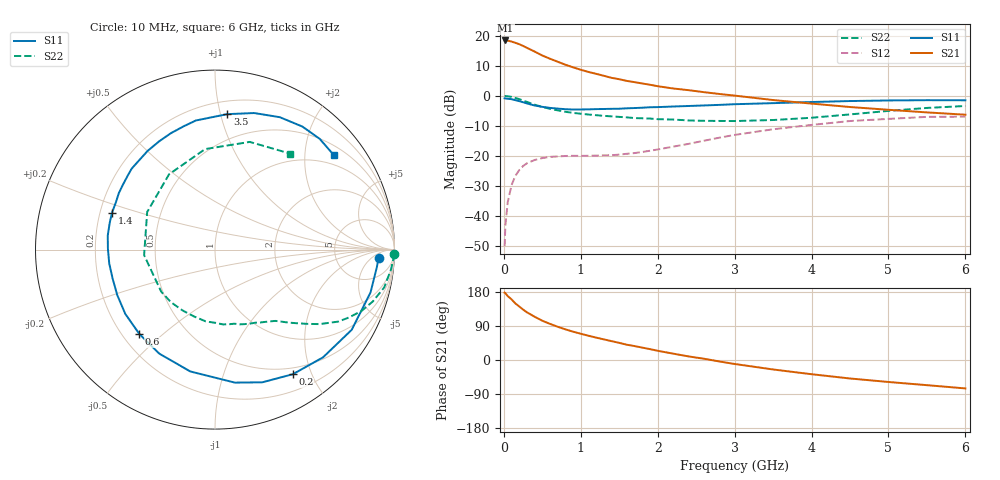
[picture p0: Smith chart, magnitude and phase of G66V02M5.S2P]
! SIEMENS Small Signal Semiconductors
! BFG193
! Si NPN RF Bipolar Junction Transistor in SOT223
! VCE = 6 V  IC = 2.5 mA
! Common Emitter S-Parameters:  August  1996
# GHz  S  MA  R  50
!  f  S11  S21  S12  S22
! GHz  MAG  ANG  MAG  ANG  MAG  ANG  MAG  ANG
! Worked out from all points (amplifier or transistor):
!   36 points, 10 MHz to 6 GHz, reference 50 ohm
!   highest |S21| = 18.5 dB at 20 MHz (marker M1)
!   |S21| within 3 dB of that: start of sweep to 343.2 MHz
!   unconditionally stable (mu >= 1): 1.33 GHz to 2.536 GHz
!   at 250 MHz: K = 0.20, MSG = 20.1 dB, |S12| = -23.4 dB
!   at 1.4 GHz: K = 1.05, MAG = 11.5 dB, |S12| = -19.8 dB
!   at 6 GHz: K = 0.93, MSG = 0.3 dB, |S12| = -6.9 dB
!   S11 on the Smith chart (normalised r, x): 10 MHz: 16, -9; 200 MHz: 0.41, -1.73; 600 MHz: 0.27, -0.42; 1.4 GHz: 0.25, +0.16; 3.5 GHz: 0.30, +1.05; 6 GHz: 0.73, +2.70
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0.01  0.9122 -3.0  8.39 177.7  0.0031 90.5  0.9957 -1.4
0.02  0.907 -6.2  8.441 176.5  0.0068 85.8  0.9962 -2.6
0.05  0.8988 -15.4  8.386 168.7  0.0167 82.0  0.9866 -6.5
0.1  0.8831 -30.4  8.094 160.0  0.0324 74.2  0.9661 -12.6
0.15  0.8501 -44.9  7.708 149.2  0.0463 65.2  0.9255 -18.2
0.2  0.8186 -58.0  7.314 141.3  0.0577 59.5  0.8853 -22.7
0.25  0.7849 -70.4  6.836 133.0  0.0675 53.3  0.8362 -26.9
0.3  0.7493 -81.5  6.356 125.9  0.075 48.5  0.7952 -30.3
0.4  0.6927 -101.5  5.51 114.2  0.0852 40.6  0.715 -35.5
0.5  0.6574 -118.2  4.731 103.6  0.0917 34.5  0.6543 -39.2
0.6  0.6314 -131.9  4.179 95.3  0.096 30.5  0.6103 -42.2
0.7  0.6149 -144.4  3.725 87.7  0.0977 27.9  0.5748 -45.0
0.8  0.6006 -155.1  3.32 80.9  0.0994 25.7  0.5438 -47.5
1.1  0.5966 179.6  2.515 64.0  0.1002 24.3  0.4891 -55.5
1.4  0.6094 160.3  2.005 49.8  0.1023 26.3  0.4562 -64.7
1.6  0.6217 149.4  1.781 40.3  0.1082 29.2  0.4383 -71.8
2.2  0.6658 124.3  1.332 16.8  0.1422 34.5  0.4034 -97.3
2.8  0.7089 104.2  1.079 -3.8  0.2006 30.9  0.3823 -129.9
3.5  0.7578 84.8  0.854 -25.0  0.2775 16.9  0.3961 -175.5
4.5  0.8214 63.9  0.653 -48.8  0.3811 -6.4  0.4913 121.4
5.5  0.8492 46.6  0.531 -66.4  0.4471 -35.1  0.6305 72.1
6  0.846 38.3  0.486 -75.0  0.4508 -50.6  0.6795 51.9
